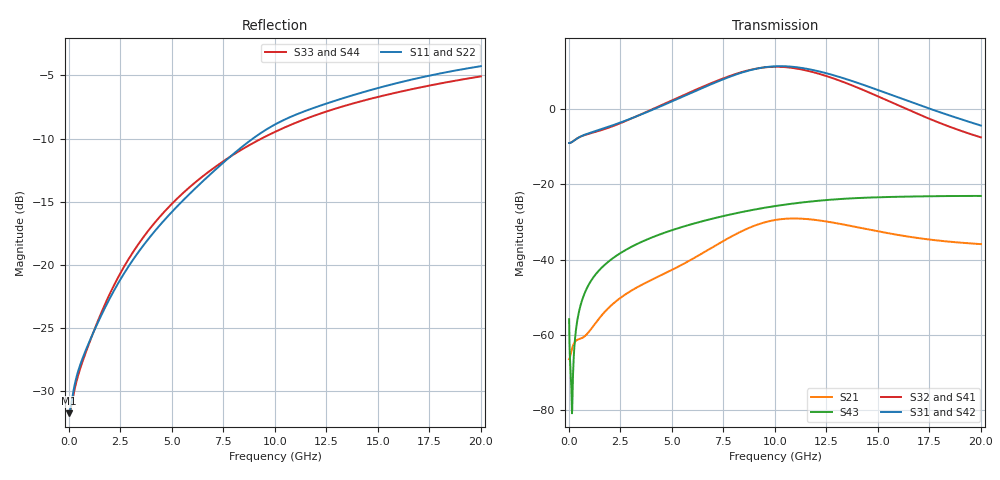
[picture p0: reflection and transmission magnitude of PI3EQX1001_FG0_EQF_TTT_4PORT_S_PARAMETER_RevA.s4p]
! NPort=4 DATA=2000 NOISE=0 GROUPDELAY=0 COMPLEX_DATAFORMAT=POLAR
! NumOfBlock=1 NumOfParam=0
! .MODEL Smodel S TSTONEFILE=PI3EQX1001_FG0_EQF_TTT_4PORT_S_PARAMETER_RevA.s4p TYPE=S
!  -- The above .MODEL line can be used for the S element in the netlist.
! The s parameter is extracted from the linear redriver, it is not bi-directional; only s(4,1)s(4,2) and s(3,1)s(3,2)
! should be the insertion loss
!Port definition:
!Port1 = input+
!Port2 = input¨C
!Port3 = output+
!Port4 = output-
# Hz S MA R  50
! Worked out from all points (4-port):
!   2000 points, 10 MHz to 20 GHz, reference 50 ohm
!   strongest paths, dB at 10 MHz, 5.01 GHz, 10.01 GHz, 15.01 GHz, 20 GHz:
!     S31: -9.0, 2.1, 11.4, 5.0, -4.4
!     S42: -9.0, 2.0, 11.3, 5.0, -4.4
!     S32: -9.0, 2.3, 11.2, 3.4, -7.5
!     S41: -9.0, 2.3, 11.2, 3.3, -7.5
!     S43: -55.8, -32.1, -25.8, -23.4, -23.1
!     S21: -66.4, -42.7, -29.5, -32.5, -35.9
!   lowest |S11| = -31.7 dB at 10 MHz (marker M1), VSWR 1.05, Z = 47.5 - j0.063 ohm
!   |S11| at or under -10 dB: start of sweep to 8.929 GHz
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1e7  0.0259 -178.5  0.0004902 2.7  3.669e-05 -0.2  4.787e-05 -0.1
     0.000479 2.9  0.02597 -178.7  4.577e-05 -0.2  5.994e-05 -0.1
     0.3546 -0.1  0.3546 179.9  0.02616 178.4  0.001616 -59.1
     0.3544 179.9  0.3545 -0.1  0.001626 -59.0  0.02613 178.4
7.13e9  0.239 -105.3  0.01485 88.5  2.177e-05 -31.0  3.196e-05 -29.7
        0.01552 86.5  0.2371 -105.3  2.889e-05 -25.6  4.015e-05 -24.9
        2.265 -54.3  2.336 130.6  0.2451 -111.8  0.03599 56.6
        2.325 130.6  2.258 -54.3  0.03599 56.6  0.245 -111.8
9.2e9  0.3278 -108.3  0.02857 60.4  1.959e-05 -27.9  3.286e-05 -32.7
       0.02956 58.9  0.3256 -108.3  3.066e-05 -25.7  3.804e-05 -24.5
       3.474 -112.6  3.481 72.4  0.3117 -114.7  0.04744 44.0
       3.461 72.5  3.465 -112.5  0.04739 43.9  0.3116 -114.6
1.101e10  0.393 -113.7  0.03415 24.8  2.188e-05 -21.0  3.469e-05 -44.7
          0.03529 23.6  0.39 -113.8  3.293e-05 -37.2  4.009e-05 -22.8
          3.604 -172.8  3.464 12.7  0.3652 -117.8  0.0564 31.6
          3.441 12.9  3.595 -172.8  0.05626 31.5  0.365 -117.7
1.345e10  0.4606 -119.1  0.0279 -8.9  2.982e-05 -37.3  3.045e-05 -69.3
          0.02893 -9.9  0.4568 -119.1  2.85e-05 -60.1  4.712e-05 -34.5
          2.505 116.3  2.217 -56.1  0.4276 -122.0  0.06486 14.4
          2.2 -55.8  2.498 116.4  0.06469 14.4  0.4275 -122.0
1.593e10  0.5243 -123.5  0.02056 -23.3  2.968e-05 -70.6  2.182e-05 -100.3
          0.02145 -24.5  0.5199 -123.6  1.915e-05 -87.4  4.425e-05 -57.7
          1.445 61.2  1.137 -106.1  0.4815 -125.8  0.06859 -1.4
          1.128 -105.6  1.441 61.3  0.06848 -1.4  0.4812 -125.7
2e10  0.6116 -130.6  0.01549 -27.6  1.679e-05 -145.0  1.463e-05 148.6
      0.01612 -29.7  0.6061 -130.6  1.015e-05 135.2  1.993e-05 -97.6
      0.6041 -4.1  0.4209 -152.1  0.5572 -131.2  0.07034 -23.8
      0.4194 -151.1  0.6019 -4.0  0.07029 -23.8  0.5571 -131.1
